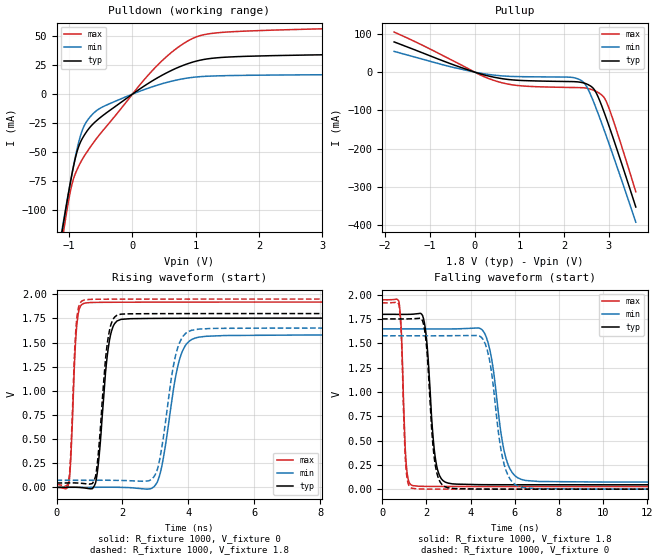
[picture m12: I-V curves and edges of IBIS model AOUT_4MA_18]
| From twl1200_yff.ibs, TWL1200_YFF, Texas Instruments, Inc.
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[Model]   AOUT_4MA_18
Model_type  Output
Vref =   1.8
Rref =   1M
Cref =   15p
Vmeas =   0.9
| variable   typ   min   max
C_comp   3.59pF   2.61pF   4.53pF
| C_pullup   3.80pF   2.61pF   4.53pF
| C_pulldown   3.39pF   2.86pF   3.95pF
[Temperature Range]   40   100   -40
| Ambient temperature   25   85   -40
[Voltage range]   1.8   1.65   1.95
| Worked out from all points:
|   slope of the pulldown table from 0 to 0.27 V, typ, clamps not added: 27.1 ohm
|   slope of the pullup table from 0 to 0.27 V, typ, clamps not added: 29.8 ohm
|   rising waveform, R_fixture 1000, V_fixture 0: 20-80 % time 255ps typ, 439ps min, 139ps max; typ from 0 V to 1.75 V
|   falling waveform, R_fixture 1000, V_fixture 1.8: 20-80 % time 318ps typ, 566ps min, 169ps max; typ from 1.8 V to 0.045 V
|   rising waveform, R_fixture 1000, V_fixture 1.8: 20-80 % time 246ps typ, 411ps min, 135ps max; typ from 0.045 V to 1.8 V
|   falling waveform, R_fixture 1000, V_fixture 0: 20-80 % time 310ps typ, 546ps min, 160ps max; typ from 1.75 V to 0 V
[Pulldown]
| AOUT_4MA_18
|   Voltage   I(typ)   I(min)   I(max)
-1.8V     -367.8mA   -352.4mA   -393.4mA
-1.105V   -116.2mA   -114.4mA   -124.4mA
-1.08V    -107.8mA   -106.4mA   -115.5mA
-970mV    -73.05mA   -72.7mA    -81.1mA
-875mV    -49.51mA   -47.17mA   -65.1mA
-785mV    -37.59mA   -30.08mA   -55.54mA
-660mV    -27.87mA   -19.08mA   -45.23mA
-465mV    -18.35mA   -10.87mA   -31.3mA
275mV     10.11mA    5.62mA     18.01mA
860mV     25.97mA    13.77mA    45.39mA
1.415V    31.65mA    15.84mA    53.24mA
3.6V      34.37mA    16.86mA    57.13mA
[Pullup]
| AOUT_4MA_18
|   Voltage   I(typ)   I(min)   I(max)
-1.8V     78.87mA    54.11mA    104.5mA
-325mV    12.96mA    8.395mA    20.11mA
505mV     -15.01mA   -8.762mA   -24.48mA
1.05V     -21.87mA   -11.9mA    -35.99mA
2.13V     -24.68mA   -13.34mA   -40.12mA
2.395V    -27.21mA   -22.98mA   -40.69mA
2.51V     -31.44mA   -39.61mA   -42.22mA
2.67V     -45.39mA   -81.64mA   -48.16mA
2.77V     -68.02mA   -112.1mA   -53.98mA
2.92V     -113.8mA   -160.3mA   -71.92mA
3.13V     -184.8mA   -230.2mA   -137.9mA
3.6V      -352.5mA   -392mA     -312.6mA
[Ramp]
| AOUT_4MA_18
| variable   typ   min   max
dV/dt_r   1.06/2.64E-10   0.96/4.50E-10   1.16/1.44E-10
dV/dt_f   1.06/3.29E-10   0.95/5.75E-10   1.16/1.79E-10
R_load = 1000
[Rising Waveform]
| AOUT_4MA_18
R_fixture =   1000
C_fixture =   0
L_fixture =   0
V_fixture =   0
V_fixture_min = 0
V_fixture_max = 0
|   Time   V(typ)   V(min)   V(max)
0s        7.719nV    38.74nV    738.7pV
390ps     887uV      -1.36uV    83.71mV
670ps     -589.5uV   -25uV      1.82V
1.085ns   -14.44mV   22.78uV    1.915V
1.64ns    1.58V      1.062mV    1.917V
2.25ns    1.747V     -3.663mV   1.917V
3.075ns   1.75V      67.29mV    1.918V
3.9ns     1.751V     1.463V     1.918V
5.115ns   1.752V     1.572V     1.919V
238ns     1.753V     1.579V     1.919V
[Falling Waveform]
| AOUT_4MA_18
R_fixture =   1000
C_fixture =   0
L_fixture =   0
V_fixture =   1.8
V_fixture_min = 1.65
V_fixture_max = 1.95
|   Time   V(typ)   V(min)   V(max)
0s        1.8V       1.65V      1.95V
760ps     1.799V     1.65V      1.936V
1.125ns   1.8V       1.65V      184.2mV
1.66ns    1.808V     1.65V      30.04mV
2.485ns   224mV      1.649V     28.13mV
3.385ns   51.65mV    1.65V      27.72mV
4.635ns   46.18mV    1.605V     27.52mV
5.685ns   45.53mV    260.3mV    27.46mV
7.105ns   45.25mV    78.9mV     27.42mV
238ns     45.1mV     72.71mV    27.4mV
[Rising Waveform]
| AOUT_4MA_18
R_fixture =   1000
C_fixture =   0
L_fixture =   0
V_fixture =   1.8
V_fixture_min = 1.65
V_fixture_max = 1.95
|   Time   V(typ)   V(min)   V(max)
0s        45.1mV     72.71mV    27.4mV
390ps     45.85mV    72.71mV    128.7mV
655ps     44.23mV    72.69mV    1.843V
1.075ns   37.58mV    72.75mV    1.947V
1.61ns    1.63V      73.05mV    1.949V
2.14ns    1.797V     69.59mV    1.949V
3.045ns   1.799V     170mV      1.95V
3.8ns     1.799V     1.544V     1.95V
4.785ns   1.8V       1.646V     1.95V
238ns     1.8V       1.65V      1.95V
[Falling Waveform]
| AOUT_4MA_18
R_fixture =   1000
C_fixture =   0
L_fixture =   0
V_fixture =   0
V_fixture_min = 0
V_fixture_max = 0
|   Time   V(typ)   V(min)   V(max)
0s        1.753V     1.579V     1.919V
760ps     1.752V     1.579V     1.904V
1.11ns    1.753V     1.579V     151.1mV
1.625ns   1.758V     1.579V     2.216mV
2.46ns    184.7mV    1.579V     621.3uV
3.305ns   6.027mV    1.58V      299.9uV
4.605ns   896.1uV    1.527V     112.9uV
5.6ns     397.7uV    195.3mV    56.81uV
6.925ns   160.8uV    5.486mV    23.5uV
238ns     18.19nV    44.04nV    8.151nV
